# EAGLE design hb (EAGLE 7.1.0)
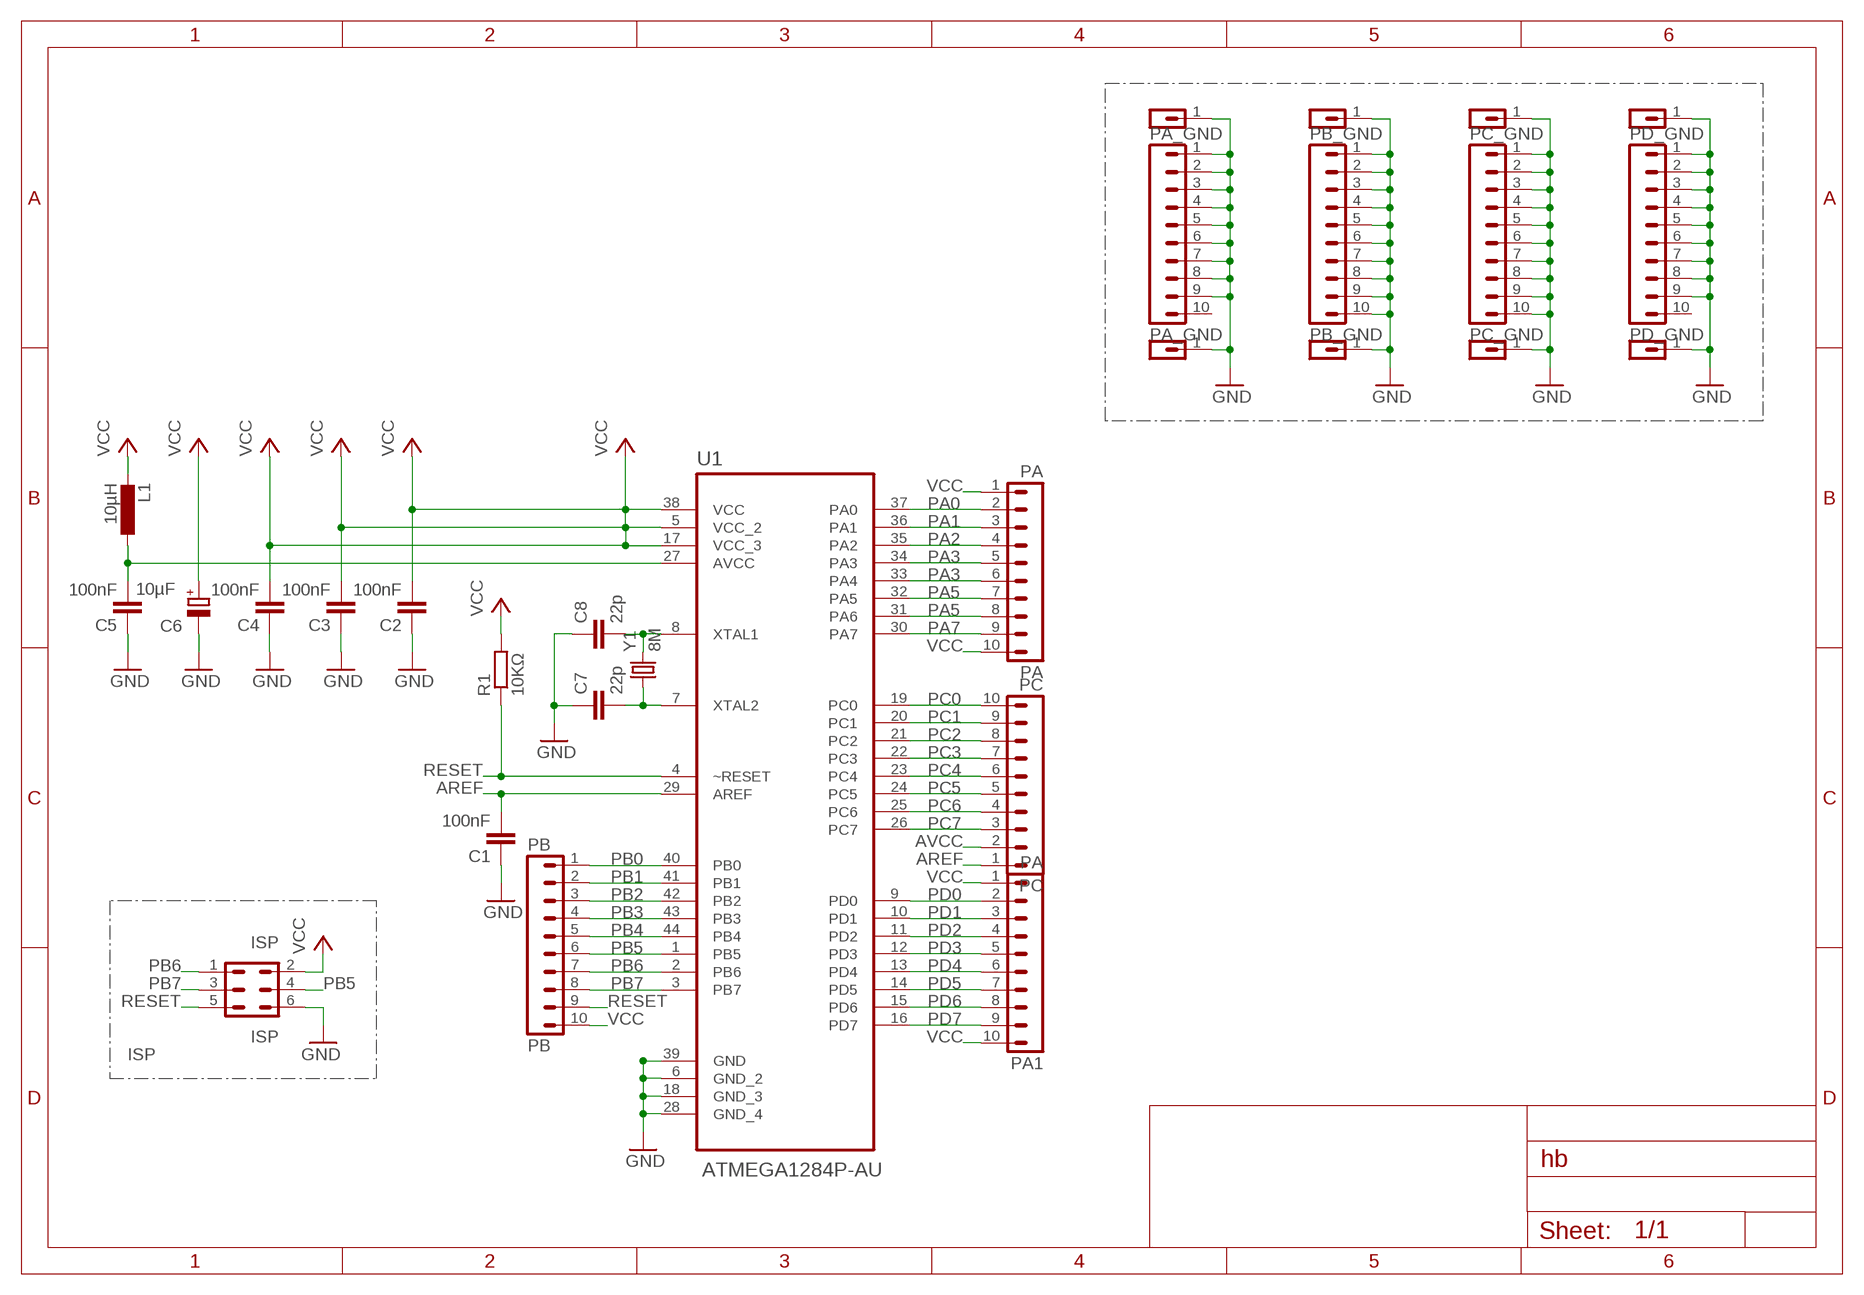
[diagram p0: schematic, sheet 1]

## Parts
C1  100nF  C-EUC0805  [C0805]
C2  100nF  C-EUC0805  [C0805]
C3  100nF  C-EUC0805  [C0805]
C4  100nF  C-EUC0805  [C0805]
C5  100nF  C-EUC0805  [C0805]
C6  10µF  CPOL-EUB  [PANASONIC_B]
C7  22p  C-EUC0805  [C0805]
C8  22p  C-EUC0805  [C0805]
ISP  ISP  MA03-2  [MA03-2]
L1  10µH  L-EUL3225P  [L3225P]
PA  PA  MA10-1  [MA10-1]
PA1  PA  MA10-1  [MA10-1]
PA_GND  PA_GND  MA10-1  [MA10-1]
PA_GND2  PA_GND  MA01-1  [MA01-1]
PA_GND3  PA_GND  MA01-1  [MA01-1]
PB  PB  MA10-1  [MA10-1]
PB_GND  PB_GND  MA10-1  [MA10-1]
PB_GND2  PB_GND  MA01-1  [MA01-1]
PB_GND3  PB_GND  MA01-1  [MA01-1]
PC  PC  MA10-1  [MA10-1]
PC_GND  PC_GND  MA10-1  [MA10-1]
PC_GND2  PC_GND  MA01-1  [MA01-1]
PC_GND3  PC_GND  MA01-1  [MA01-1]
PD_GND  PD_GND  MA10-1  [MA10-1]
PD_GND2  PD_GND  MA01-1  [MA01-1]
PD_GND3  PD_GND  MA01-1  [MA01-1]
R1  10KΩ  R-EU_R0805  [R0805]
U1  ATMEGA1284P-AU  [QFP80P1200X1200X120-44N]
Y1  8M  CRYSTAL5X3  [CRYSTAL-SMD-5X3]

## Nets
AREF: C1.2 PC.1 U1.29(AREF)
AVCC: C5.2 L1.1 PC.2 U1.27(AVCC)
GND: C1.1 C2.1 C3.1 C4.1 C5.1 C6.- C7.1 C8.1 ISP.6 PA_GND2.1 PA_GND3.1 PA_GND.1 PA_GND.2 PA_GND.3 PA_GND.4 PA_GND.5 PA_GND.6 PA_GND.7 PA_GND.8 PA_GND.9 PB_GND2.1 PB_GND3.1 PB_GND.1 PB_GND.2 PB_GND.3 PB_GND.4 PB_GND.5 PB_GND.6 PB_GND.7 PB_GND.8 PB_GND.9 PB_GND.10 PC_GND2.1 PC_GND3.1 PC_GND.1 PC_GND.2 PC_GND.3 PC_GND.4 PC_GND.5 PC_GND.6 PC_GND.7 PC_GND.8 PC_GND.9 PC_GND.10 PD_GND2.1 PD_GND3.1 PD_GND.1 PD_GND.2 PD_GND.3 PD_GND.4 PD_GND.5 PD_GND.6 PD_GND.7 PD_GND.8 PD_GND.9 U1.6(GND_2) U1.18(GND_3) U1.28(GND_4) U1.39(GND)
PA0: PA.2 U1.37(PA0)
PA1: PA.3 U1.36(PA1)
PA2: PA.4 U1.35(PA2)
PA3: PA.5 U1.34(PA3)
PA4: PA.6 U1.33(PA4)
PA5: PA.7 U1.32(PA5)
PA6: PA.8 U1.31(PA6)
PA7: PA.9 U1.30(PA7)
PB0: PB.1 U1.40(PB0)
PB1: PB.2 U1.41(PB1)
PB2: PB.3 U1.42(PB2)
PB3: PB.4 U1.43(PB3)
PB4: PB.5 U1.44(PB4)
PB5: ISP.4 PB.6 U1.1(PB5)
PB6: ISP.1 PB.7 U1.2(PB6)
PB7: ISP.3 PB.8 U1.3(PB7)
PC0: PC.10 U1.19(PC0)
PC1: PC.9 U1.20(PC1)
PC2: PC.8 U1.21(PC2)
PC3: PC.7 U1.22(PC3)
PC4: PC.6 U1.23(PC4)
PC5: PC.5 U1.24(PC5)
PC6: PC.4 U1.25(PC6)
PC7: PC.3 U1.26(PC7)
PD0: PA1.2 U1.9(PD0)
PD1: PA1.3 U1.10(PD1)
PD2: PA1.4 U1.11(PD2)
PD3: PA1.5 U1.12(PD3)
PD4: PA1.6 U1.13(PD4)
PD5: PA1.7 U1.14(PD5)
PD6: PA1.8 U1.15(PD6)
PD7: PA1.9 U1.16(PD7)
RESET: ISP.5 PB.9 R1.1 U1.4(~RESET)
VCC: C2.2 C3.2 C4.2 C6.+ ISP.2 L1.2 PA1.1 PA1.10 PA.1 PA.10 PB.10 R1.2 U1.5(VCC_2) U1.17(VCC_3) U1.38(VCC)
XTAL1: C8.2 U1.8(XTAL1) Y1.3
XTAL2: C7.2 U1.7(XTAL2) Y1.1
Unconnected: PA_GND.10 PD_GND.10

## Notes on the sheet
- ISP

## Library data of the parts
C1-C5 C7 C8 = rcl:C-EU: CAPACITOR, European symbol
C6 = rcl:CPOL-EU: POLARIZED CAPACITOR, European symbol
ISP = con-lstb_1:MA03-2: PIN HEADER; OC_FARNELL: unknown; OC_NEWARK: unknown
L1 = rcl:L-EU: INDUCTOR, European symbol
PA PA1 PA_GND PB PB_GND PC PC_GND PD_GND = con-lstb_1:MA10-1: PIN HEADER; OC_FARNELL: unknown; OC_NEWARK: unknown
PA_GND2 PA_GND3 PB_GND2 PB_GND3 PC_GND2 PC_GND3 PD_GND2 PD_GND3 = con-lstb_1:MA01-1
R1 = rcl:R-EU_: RESISTOR, European symbol
U1 = Atmel_By_element14_Batch_1-00:ATMEGA1284P-AU: Microcontroller with Programmable Flash; MPN: ATMEGA1284P-AU; OC_FARNELL: 1715480; OC_NEWARK: 15R0263; PACKAGE: TQFP-44; SUPPLIER: Atmel
Y1 = SparkFun-FreqCtrl:CRYSTAL: Various standard crystals. Proven footprints. Spark Fun Electronics SKU : COM-00534

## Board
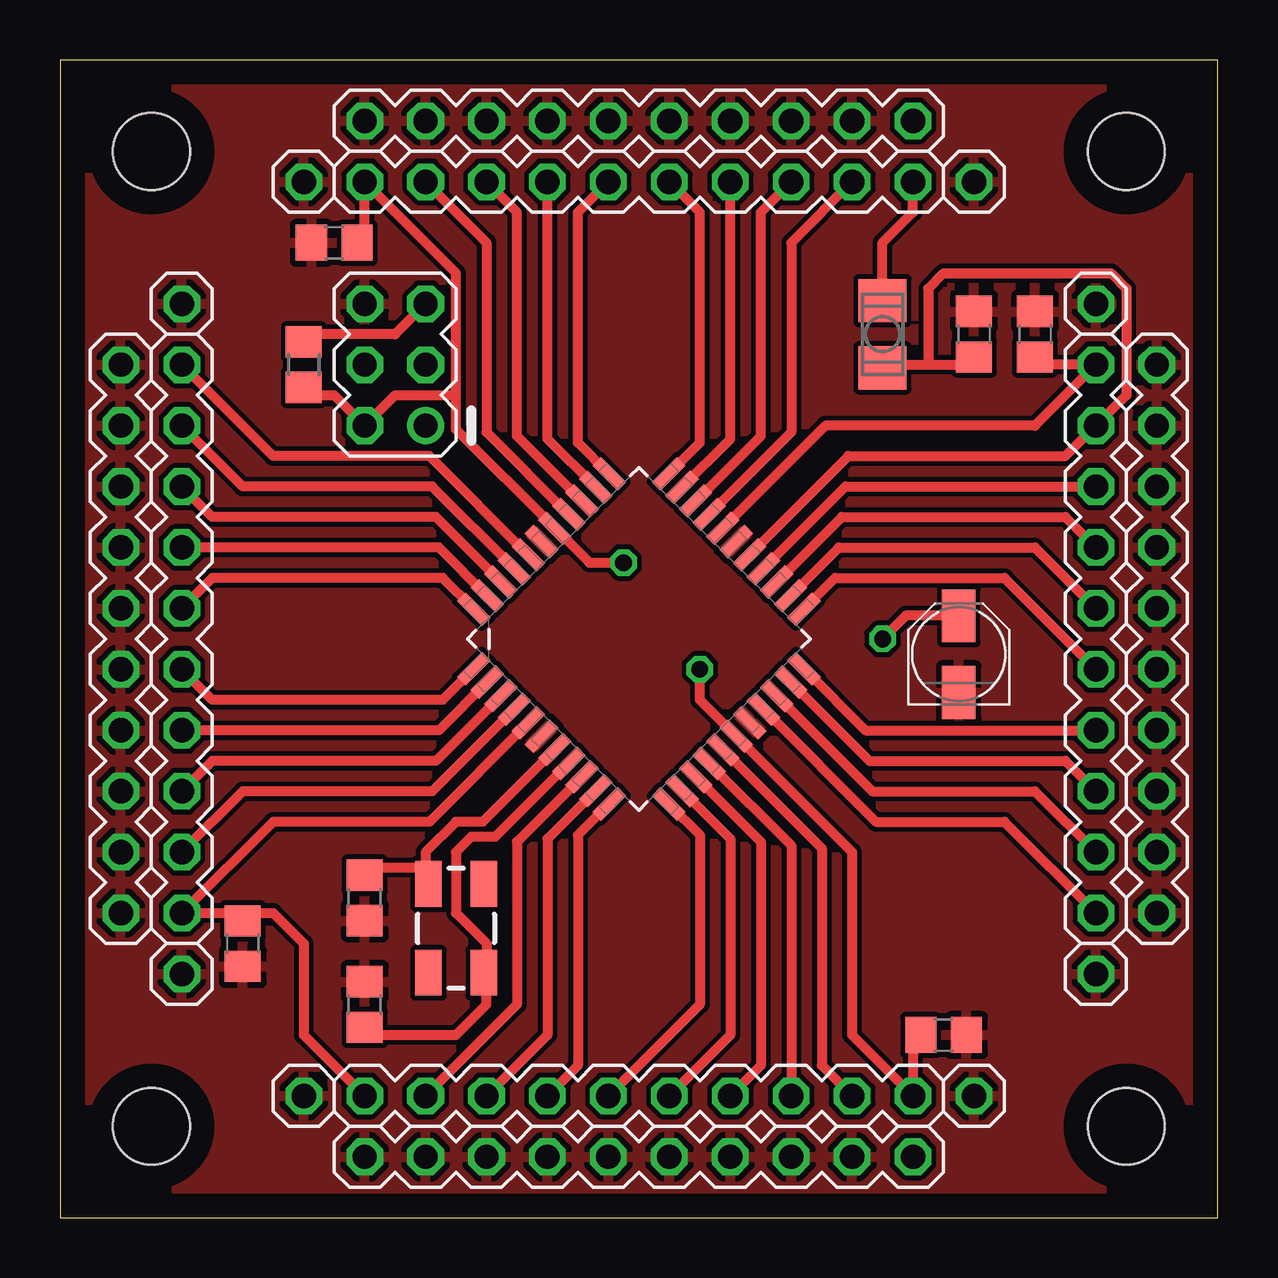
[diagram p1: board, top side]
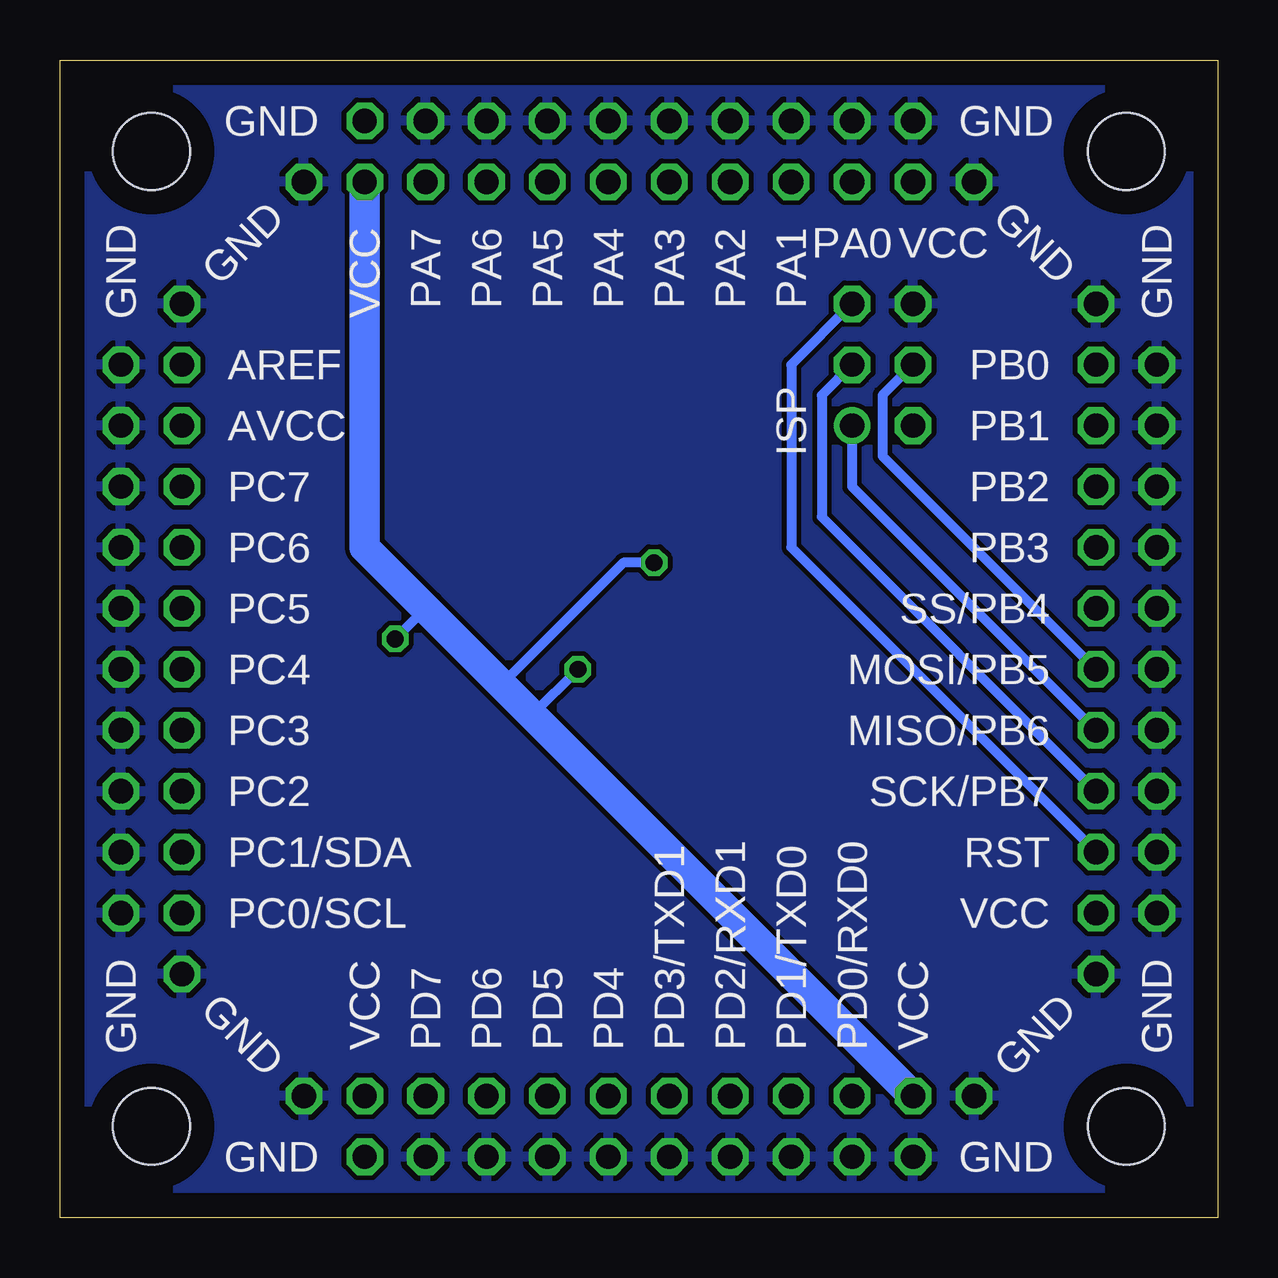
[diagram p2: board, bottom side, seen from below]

Size 48.26 x 48.26 mm. Coordinates in mm from the lower left corner, seen from the top.
Outline: 0,0 48.26,0 48.26,48.26 0,48.26 0,0
Copper layers (1*16): Top 0.035mm / dielectric 1.5mm / Bottom 0.035mm
Design rules "default": minimum track width 10mil, minimum drill 24mil, track to track 8mil, track to pad 8mil, pad to pad 8mil, via to via 8mil, smd to smd 8mil, copper to edge 40mil, drill to drill 8mil, minimum pad ring 10mil, minimum via ring 8mil, stop-mask expansion 4mil, vias tented up to drill 0mil, thermal gap 10mil
Holes 3.2 mm at 3.81,3.81 3.81,44.45 44.45,44.45 44.45,3.81

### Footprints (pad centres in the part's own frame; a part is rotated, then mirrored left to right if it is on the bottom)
C0805 = smd 1.3 x 1.5: 1 -0.95,0; 2 0.95,0
PANASONIC_B = smd 2.2 x 1.4: + 1.6,0; - -1.6,0
MA03-2 = drill 1.016: 1 -2.54,-1.27 | drill 1.016 octagon: 2 -2.54,1.27; 3 0,-1.27; 4 0,1.27; 5 2.54,-1.27; 6 2.54,1.27
L3225P = smd 1.8 x 2: 1 -1.4,0; 2 1.4,0
MA10-1 = drill 1.016 octagon: 1 -11.43,0; 2 -8.89,0; 3 -6.35,0; 4 -3.81,0; 5 -1.27,0; 6 1.27,0; 7 3.81,0; 8 6.35,0; 9 8.89,0; 10 11.43,0
MA01-1 = drill 1.016 octagon: 1 0,0
R0805 = smd 1.3 x 1.5: 1 -0.95,0; 2 0.95,0
QFP80P1200X1200X120-44N = smd 1.473 x 0.508: 1 -5.74,3.988; 2 -5.74,3.2; 3 -5.74,2.388; 4 -5.74,1.6; 5 -5.74,0.787; 6 -5.74,0; 7 -5.74,-0.787; 8 -5.74,-1.6; 9 -5.74,-2.388; 10 -5.74,-3.2; 11 -5.74,-3.988; 23 5.74,-3.988; 24 5.74,-3.2; 25 5.74,-2.388; 26 5.74,-1.6; 27 5.74,-0.787; 28 5.74,0; 29 5.74,0.787; 30 5.74,1.6; 31 5.74,2.388; 32 5.74,3.2; 33 5.74,3.988 | smd 0.508 x 1.473: 12 -3.988,-5.74; 13 -3.2,-5.74; 14 -2.388,-5.74; 15 -1.6,-5.74; 16 -0.787,-5.74; 17 0,-5.74; 18 0.787,-5.74; 19 1.6,-5.74; 20 2.388,-5.74; 21 3.2,-5.74; 22 3.988,-5.74; 34 3.988,5.74; 35 3.2,5.74; 36 2.388,5.74; 37 1.6,5.74; 38 0.787,5.74; 39 0,5.74; 40 -0.787,5.74; 41 -1.6,5.74; 42 -2.388,5.74; 43 -3.2,5.74; 44 -3.988,5.74
CRYSTAL-SMD-5X3 = smd 1.9 x 1.1: 1 -1.85,-1.15; 2 1.85,-1.15; 3 1.85,1.15; 4 -1.85,1.15

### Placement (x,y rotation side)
C1  40.64,36.83 270 top
C2  7.62,11.43 90 top
C3  36.83,7.62 180 top
C4  11.43,40.64 0 top
C5  38.1,36.83 270 top
C6  37.47,23.5 90 top
C7  12.7,13.34 90 top
C8  12.7,8.89 270 top
ISP  13.97,35.56 90 top
L1  34.29,36.83 90 top
PA  24.13,43.18 0 top
PA1  24.13,5.08 0 top
PA_GND  24.13,45.72 0 top
PA_GND2  10.16,43.18 0 top
PA_GND3  38.1,43.18 0 top
PB  5.08,24.13 270 top
PB_GND  2.54,24.13 270 top
PB_GND2  5.08,38.1 90 top
PB_GND3  5.08,10.16 90 top
PC  43.18,24.13 270 top
PC_GND  45.72,24.13 270 top
PC_GND2  43.18,38.1 90 top
PC_GND3  43.18,10.16 90 top
PD_GND  24.13,2.54 0 top
PD_GND2  10.16,5.08 0 top
PD_GND3  38.1,5.08 270 top
R1  10.16,35.56 270 top
U1  24.13,24.13 45 top
Y1  16.51,12.06 270 top

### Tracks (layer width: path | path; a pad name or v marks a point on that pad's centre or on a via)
AREF
  Top 0.406: U1.29 31.91,33.02 40.64,33.02 PC.1 40.64,35.56 C1.2
AVCC
  Top 0.406: U1.27 32.86,31.75 41.91,31.75 PC.2 44.45,34.29 44.45,38.73 43.81,39.37 36.83,39.37 36.2,38.73 36.2,35.56 | 34.29,35.56 L1.1 34.42,35.56 36.2,35.56 | C5.2 37.78,35.56 36.2,35.56
GND
  pour Top: -2.54,-2.54 50.8,-2.54 50.8,50.8 -2.54,50.8
  pour Bottom: -1.27,49.53 49.53,49.53 49.53,-1.44 0.17,-1.44 -1.27,-1.27
PA0
  Top 0.406: U1.37 17.78,32.74 17.78,40.64 PA.2
PA1
  Top 0.406: U1.36 19.05,32.59 19.05,41.91 PA.3
PA2
  Top 0.406: U1.35 20.32,32.47 PA.4
PA3
  Top 0.406: U1.34 21.59,32.31 21.59,41.91 PA.5
PA4
  Top 0.406: U1.33 26.67,32.31 26.67,41.91 PA.6
PA5
  Top 0.406: U1.32 27.94,32.47 PA.7
PA6
  Top 0.406: U1.31 29.21,32.59 29.21,41.91 PA.8
PA7
  Top 0.406: PA.9 30.48,40.64 30.48,32.74 U1.30
PB0
  Top 0.406: U1.40 15.4,31.75 8.89,31.75 PB.1
PB1
  Top 0.406: U1.41 15.52,30.48 7.62,30.48 PB.2
PB2
  Top 0.406: U1.42 15.67,29.21 6.35,29.21 PB.3
PB3
  Top 0.406: U1.43 15.79,27.94 PB.4
PB4
  Top 0.406: U1.44 15.95,26.67 6.35,26.67 PB.5
PB5
  Top 0.406: U1.1 15.95,21.59 6.35,21.59 PB.6
  Bottom 0.406: ISP.4 13.97,34.29 13.97,31.75 PB.6
PB6
  Top 0.406: U1.2 15.79,20.32 PB.7
  Bottom 0.406: ISP.1 15.24,30.48 PB.7
PB7
  Top 0.406: U1.3 15.67,19.05 6.35,19.05 PB.8
  Bottom 0.406: ISP.3 16.51,34.29 16.51,29.21 PB.8
PC0
  Top 0.406: U1.19 34.01,16.51 39.37,16.51 PC.10
PC1
  Top 0.406: U1.20 33.86,17.78 40.64,17.78 PC.9
PC2
  Top 0.406: U1.21 33.74,19.05 41.91,19.05 PC.8
PC3
  Top 0.406: U1.22 33.58,20.32 PC.7
PC4
  Top 0.406: U1.23 32.31,26.67 39.37,26.67 PC.6
PC5
  Top 0.406: U1.24 32.47,27.94 40.64,27.94 PC.5
PC6
  Top 0.406: U1.25 32.59,29.21 41.91,29.21 PC.4
PC7
  Top 0.406: U1.26 32.74,30.48 PC.3
PD0
  Top 0.406: U1.9 19.05,15.67 19.05,8.89 PA1.2
PD1
  Top 0.406: U1.10 20.32,15.79 20.32,7.62 PA1.3
PD2
  Top 0.406: U1.11 21.59,15.95 21.59,6.35 PA1.4
PD3
  Top 0.406: U1.12 26.67,15.95 26.67,8.89 PA1.5
PD4
  Top 0.406: U1.13 27.94,15.79 27.94,7.62 PA1.6
PD5
  Top 0.406: U1.14 29.21,15.67 29.21,6.35 PA1.7
PD6
  Top 0.406: U1.15 30.48,15.52 PA1.8
PD7
  Top 0.406: U1.16 31.75,15.4 31.75,6.35 PA1.9
RESET
  Top 0.406: U1.4 15.52,17.78 7.62,17.78 PB.9 | ISP.5 13.97,36.83 10.16,36.83 R1.1
  Bottom 0.406: ISP.5 17.78,35.56 17.78,27.94 PB.9
VCC  (via drill 0.7)
  Top 0.406: U1.17 | 12.7,40.96 12.7,40.64 C4.2 12.7,40.96 | U1.5 15.4,16.51 8.89,16.51 PB.10 7.62,12.7 C2.2 7.94,12.7 8.89,12.7 10.16,11.43 10.16,7.62 PA1.1 | L1.2 34.29,40.64 35.56,41.91 PA.10 | R1.2 10.48,34.29 11.43,34.29 ISP.2 13.97,34.29 16.51,34.29 | C3.2 35.56,7.62 PA1.10 33.02,7.62 33.02,15.24 U1.17 | 12.7,40.96 PA.1 16.51,39.37 16.51,34.29 | 16.51,34.29 16.51,32.86 U1.38 22.07,27.3 v23.5,27.3 | C6.+ 35.26,25.09 v34.29,24.13 | U1.17 26.67,21.59 v26.67,22.86 26.51,22.86
  Bottom 0.406: 33.02,25.4 v34.29,24.13 | v26.67,22.86 28.57,20.95 | v23.5,27.3 24.77,27.3 29.84,22.23
  Bottom 1.27: PA.10 35.56,27.94 33.02,25.4 29.84,22.23 28.57,20.95 PA1.1
XTAL1
  Top 0.406: 17.78,10.16 17.78,8.89 16.51,7.62 13.02,7.62 C8.2 | U1.8 18.14,15.88 17.14,15.88 16.51,15.24 16.51,12.7 17.78,11.43 17.78,10.16 | 17.78,10.16 17.73,10.21 | Y1.3 17.71,10.16 17.78,10.16
XTAL2
  Top 0.406: C7.2 13.02,14.61 15.24,14.61 15.36,14.48 Y1.1 15.29,13.91 15.24,13.97 15.24,15.24 16.51,16.51 17.62,16.51 U1.7

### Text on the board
bPlace: GND | GND | GND | VCC | PA0 | PA1 | PA2 | PA3 | PA4 | PA5 | PA6 | PA7 | VCC | GND | GND | GND | PB0 | AREF | PB1 | AVCC | ISP | PB2 | PC7 | PB3 | PC6 | SS/PB4 | PC5 | MOSI/PB5 | PC4 | MISO/PB6 | PC3 | SCK/PB7 | PC2 | RST | PC1/SDA | VCC | PC0/SCL | GND | GND | GND | GND | VCC | PD0/RXD0 | PD1/TXD0 | PD2/RXD1 | PD3/TXD1 | PD4 | PD5 | PD6 | PD7 | VCC | GND | GND
Vscore: C4 | L1 | R1 | C5 | C1 | C6 | C7 | Y1 | C2 | C3 | C8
